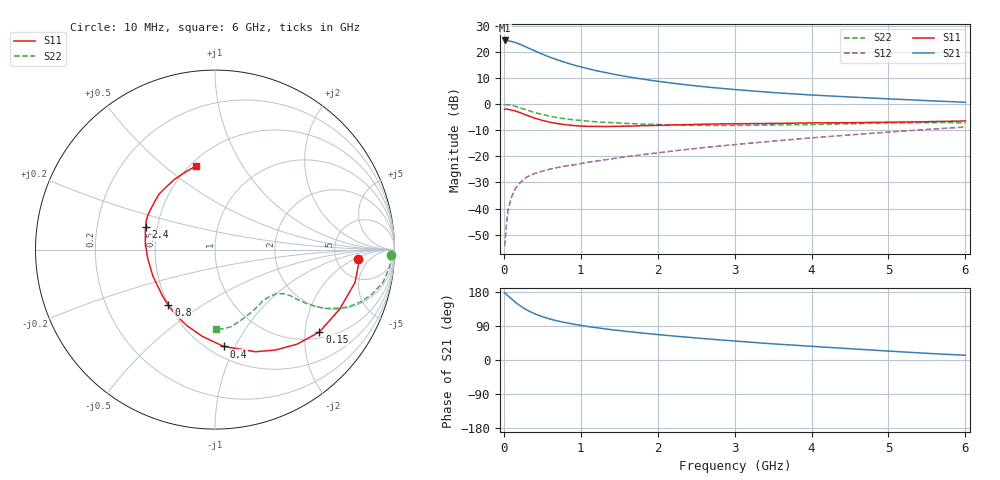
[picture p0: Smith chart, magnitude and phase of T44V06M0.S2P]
! Infineon Technologies  Discrete & RF Semiconductors
! BFR182T
! Si NPN RF Bipolar Junction Transistor in SC75
! VCE = 4 V  IC = 6 mA
! Common Emitter S-Parameters:  October  1999
# GHz  S  MA  R  50
!  f  S11  S21  S12  S22
! GHz  MAG  ANG  MAG  ANG  MAG  ANG  MAG  ANG
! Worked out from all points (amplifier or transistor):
!   36 points, 10 MHz to 6 GHz, reference 50 ohm
!   highest |S21| = 24.4 dB at 10 MHz (marker M1)
!   |S21| within 3 dB of that: start of sweep to 326.9 MHz
!   unconditionally stable (mu >= 1): 1.308 GHz to 3.961 GHz
!   at 250 MHz: K = 0.32, MSG = 25.8 dB, |S12| = -29.1 dB
!   at 1.4 GHz: K = 1.02, MAG = 15.4 dB, |S12| = -21.0 dB
!   at 6 GHz: K = 0.84, MSG = 4.7 dB, |S12| = -8.7 dB
!   lowest NFmin = 1.25 dB at 450 MHz
!   S11 on the Smith chart (normalised r, x): 10 MHz: 8.23, -2.33; 150 MHz: 1.17, -2.38; 400 MHz: 0.59, -0.90; 800 MHz: 0.50, -0.37; 2.4 GHz: 0.43, +0.13; 6 GHz: 0.54, +0.65
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0.01  0.7979 -3.7  16.68 177.1  0.0019 85.2  0.9809 -1.9
0.02  0.807 -3.9  16.65 176.2  0.0028 93.7  0.9795 -2.2
0.05  0.8011 -13.3  16.57 170.2  0.0087 87.9  0.9788 -5.7
0.1  0.7696 -25.6  15.96 161.3  0.0167 78.6  0.9531 -11.1
0.15  0.7411 -38.3  15.21 152.4  0.0241 72.1  0.9095 -15.8
0.2  0.6975 -49.1  14.31 144.7  0.0299 69.2  0.8654 -19.6
0.25  0.6535 -58.9  13.27 138.0  0.0352 63.4  0.816 -22.7
0.3  0.6121 -68.4  12.3 131.9  0.0404 61.7  0.7734 -25.0
0.4  0.5416 -84.9  10.57 121.9  0.0469 56.9  0.693 -28.2
0.5  0.489 -98.2  9.123 114.4  0.0521 55.2  0.6351 -29.6
0.6  0.4515 -110.5  7.964 108.1  0.057 54.4  0.5887 -30.6
0.7  0.4245 -120.8  7.061 103.0  0.0614 53.6  0.5525 -31.0
0.8  0.4046 -130.0  6.32 98.6  0.0652 54.5  0.5253 -31.3
0.9  0.3907 -138.3  5.698 94.8  0.0684 55.5  0.5027 -31.4
1.1  0.3762 -151.9  4.773 88.1  0.0774 56.4  0.4735 -32.0
1.6  0.38 -176.3  3.381 75.3  0.0991 59.5  0.4282 -34.8
2.2  0.3995 166.5  2.522 63.4  0.1268 61.9  0.4028 -40.5
2.4  0.4062 162.0  2.328 59.9  0.1369 62.4  0.396 -42.9
3.5  0.4283 142.4  1.672 42.6  0.1961 61.9  0.4001 -56.9
4.5  0.4423 128.2  1.375 29.8  0.2582 58.9  0.4222 -71.2
5.5  0.4625 110.9  1.172 17.6  0.3285 54.2  0.4431 -83.9
6  0.4776 102.8  1.089 12.5  0.3656 50.8  0.4422 -89.3
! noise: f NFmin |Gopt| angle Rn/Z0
0.45  1.25  0.25  39  0.3
0.9  1.4  0.25  78  0.23
1.8  1.95  0.21  151  0.2
